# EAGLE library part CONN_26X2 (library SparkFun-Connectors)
Multi connection point. Often used as Generic Header-pin footprint for 0.1 inch spaced/style header connections On any of the 0.1 inch spaced packages, you can populate with these: Break Away Headers - Straight (PRT-00116) Break Away Male Headers - Right Angle (PRT-00553) Female Headers (PRT-00115) Break Away Headers - Machine Pin (PRT-00117) Break Away Female Headers - Swiss Machine Pin (PRT-00743)
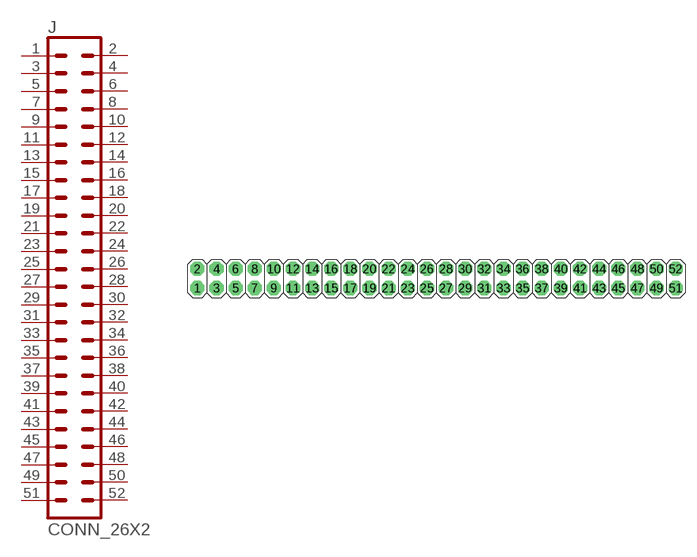
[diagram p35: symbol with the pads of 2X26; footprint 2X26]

Designator prefix J

## CONN_26X2  [2X26]
1  1  pas
2  2  pas
3  3  pas
4  4  pas
5  5  pas
6  6  pas
7  7  pas
8  8  pas
9  9  pas
10  10  pas
11  11  pas
12  12  pas
13  13  pas
14  14  pas
15  15  pas
16  16  pas
17  17  pas
18  18  pas
19  19  pas
20  20  pas
21  21  pas
22  22  pas
23  23  pas
24  24  pas
25  25  pas
26  26  pas
27  27  pas
28  28  pas
29  29  pas
30  30  pas
31  31  pas
32  32  pas
33  33  pas
34  34  pas
35  35  pas
36  36  pas
37  37  pas
38  38  pas
39  39  pas
40  40  pas
41  41  pas
42  42  pas
43  43  pas
44  44  pas
45  45  pas
46  46  pas
47  47  pas
48  48  pas
49  49  pas
50  50  pas
51  51  pas
52  52  pas

## Footprint 2X26 (pad centres in mm)
Plated Through Hole - 2x26 Specifications: Pin count:52 Pin pitch:0.1" Example device(s): CONN_26x2
drill 1.016 pad 1.88 octagon: 1 -11.43,-1.27; 2 -11.43,1.27; 3 -8.89,-1.27; 4 -8.89,1.27; 5 -6.35,-1.27; 6 -6.35,1.27; 7 -3.81,-1.27; 8 -3.81,1.27; 9 -1.27,-1.27; 10 -1.27,1.27; 11 1.27,-1.27; 12 1.27,1.27; 13 3.81,-1.27; 14 3.81,1.27; 15 6.35,-1.27; 16 6.35,1.27; 17 8.89,-1.27; 18 8.89,1.27; 19 11.43,-1.27; 20 11.43,1.27; 21 13.97,-1.27; 22 13.97,1.27; 23 16.51,-1.27; 24 16.51,1.27; 25 19.05,-1.27; 26 19.05,1.27; 27 21.59,-1.27; 28 21.59,1.27; 29 24.13,-1.27; 30 24.13,1.27; 31 26.67,-1.27; 32 26.67,1.27; 33 29.21,-1.27; 34 29.21,1.27; 35 31.75,-1.27; 36 31.75,1.27; 37 34.29,-1.27; 38 34.29,1.27; 39 36.83,-1.27; 40 36.83,1.27; 41 39.37,-1.27; 42 39.37,1.27; 43 41.91,-1.27; 44 41.91,1.27; 45 44.45,-1.27; 46 44.45,1.27; 47 46.99,-1.27; 48 46.99,1.27; 49 49.53,-1.27; 50 49.53,1.27; 51 52.07,-1.27; 52 52.07,1.27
